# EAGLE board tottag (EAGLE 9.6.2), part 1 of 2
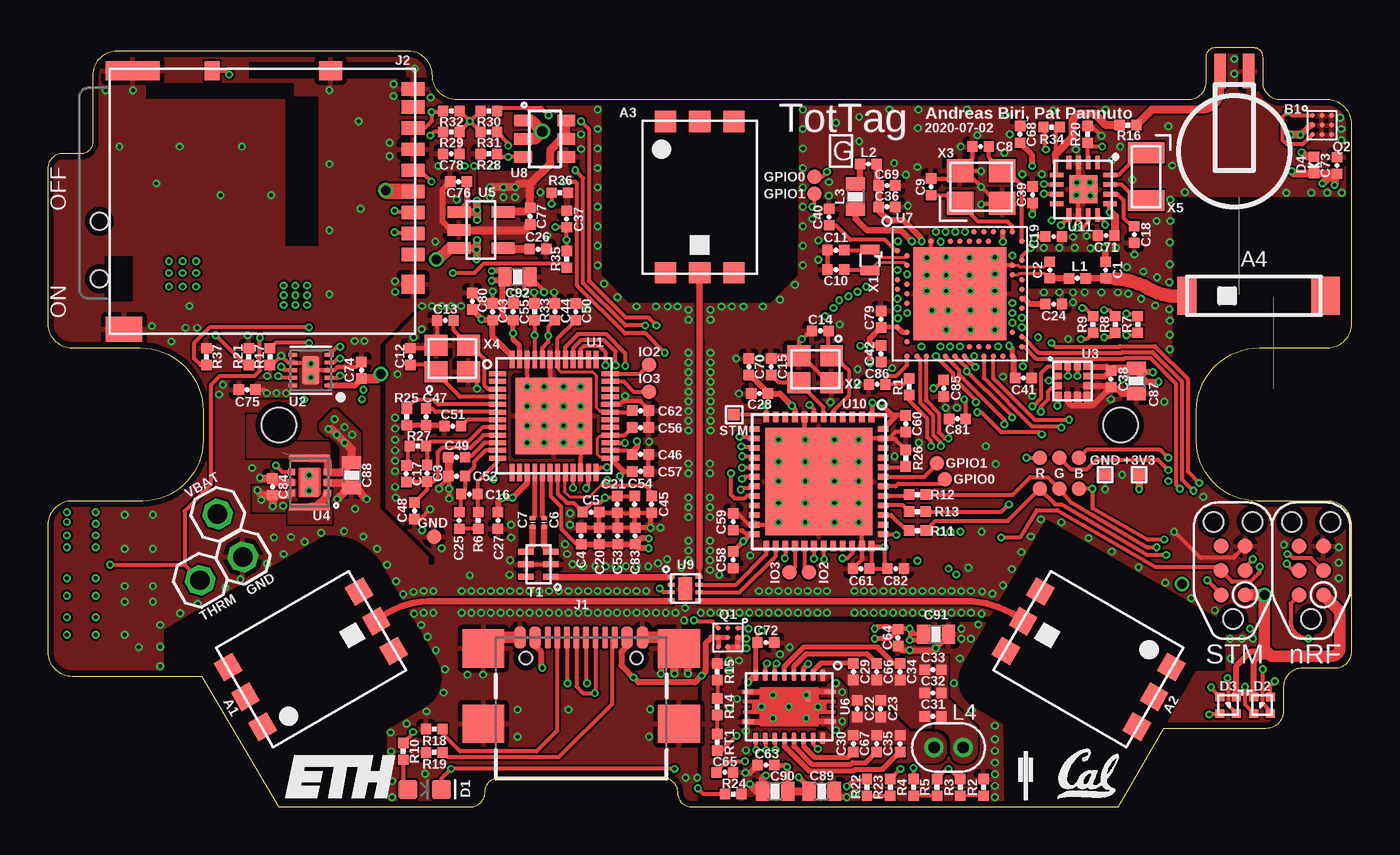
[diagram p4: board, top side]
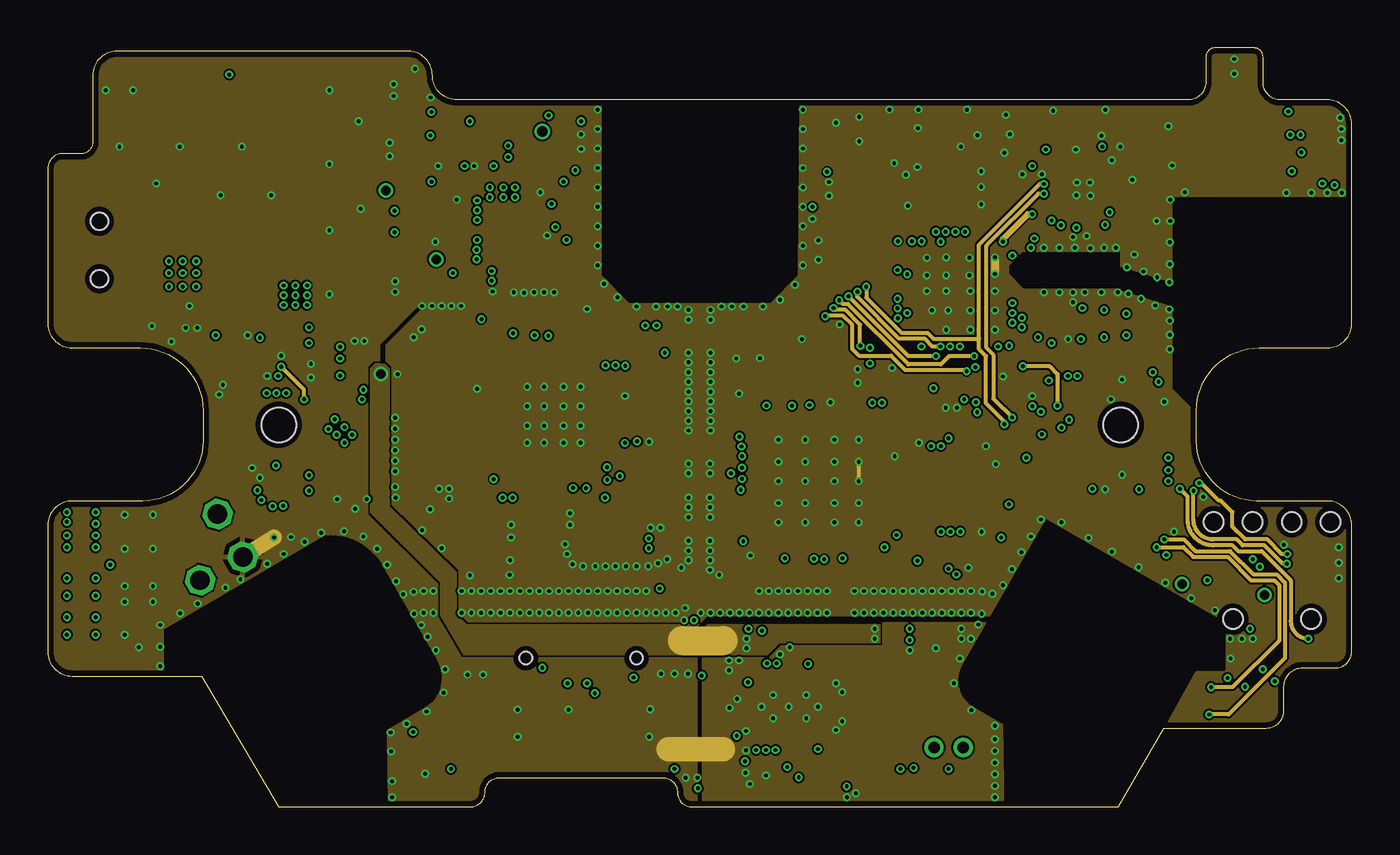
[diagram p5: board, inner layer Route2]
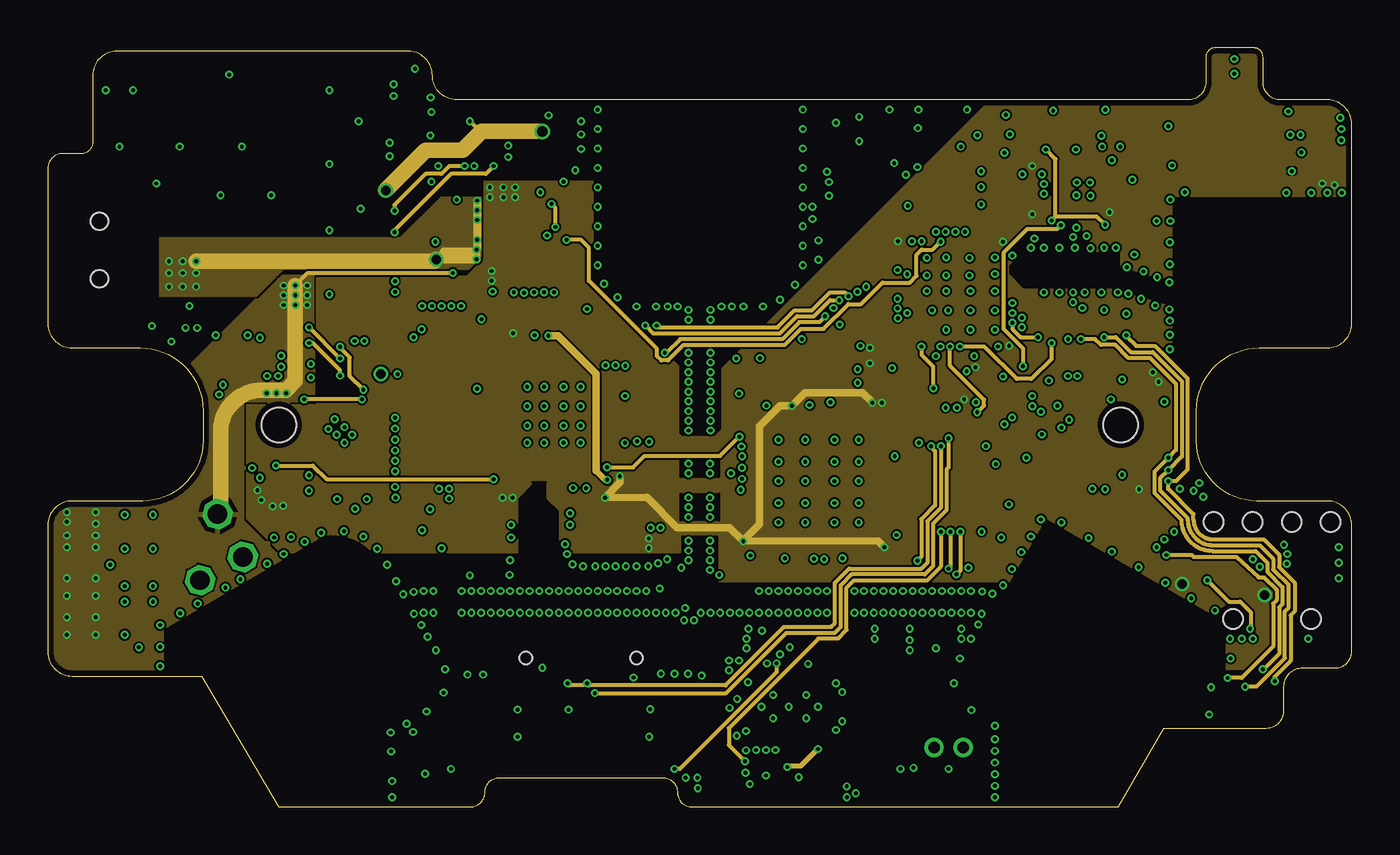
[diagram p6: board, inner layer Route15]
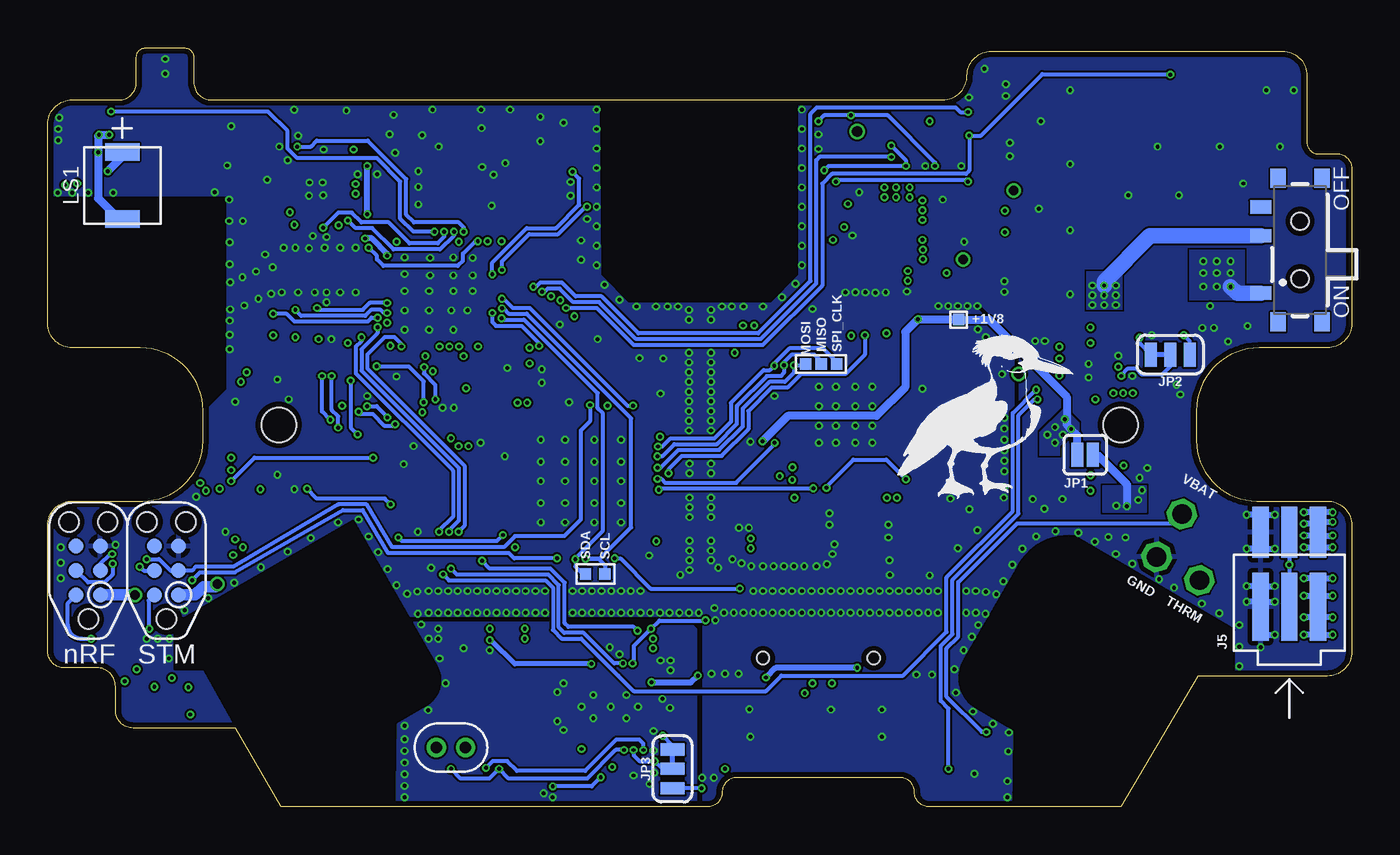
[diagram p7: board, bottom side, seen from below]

Size 68.14 x 39.65 mm. Coordinates in mm from the lower left corner, seen from the top.
Outline: 66.87,36.93 64.42,36.93 arc-90 63.51,37.85 63.51,39.17 arc90 63.02,39.65 60.99,39.65 arc90 60.51,39.17 60.51,37.85 arc-90 59.59,36.93 21.37,36.93 arc-90 20.1,38.2 arc90 18.83,39.47 3.61,39.47 arc90 2.34,38.2 2.34,34.7 arc-90 1.76,34.12 0.76,34.12 arc90 0,33.36 0,25.25 arc90 1.27,23.98 4.83,23.98 arc-90 8.11,20.69 8.11,19.14 arc-90 4.95,15.98 1.27,15.98 arc90 0,14.71 0,8.1 arc90 1.27,6.83 8.03,6.83 12.07,0 22.08,0 arc90 22.84,0.76 arc-90 23.6,1.52 32.14,1.52 arc-90 32.9,0.76 arc90 33.66,0 55.94,0 58.33,4.11 63.68,4.11 arc90 64.6,5.03 64.6,6.3 arc-90 65.56,7.26 67.29,7.26 arc90 68.14,8.11 68.14,14.71 arc90 66.87,15.98 63.18,15.98 arc-90 60.02,19.14 60.02,20.69 arc-90 63.31,23.98 66.87,23.98 arc90 68.14,25.25 68.14,35.66 arc90 66.87,36.93
Copper layers (1+2*15+16): Top 0.0356mm / dielectric 0.18mm / Route2 0.0356mm / dielectric 1.03mm / Route15 0.0356mm / dielectric 0.18mm / Bottom 0.0356mm
Design rules "quickturn_co_kr_1oz_4lyr *": minimum track width 4mil, minimum drill 8mil, track to track 4mil, track to pad 4mil, pad to pad 4mil, via to via 4mil, smd to smd 4mil, copper to edge 12mil, drill to drill 12mil, minimum pad ring 8mil, minimum via ring 4mil, stop-mask expansion 3mil, vias tented up to drill 50mil, thermal gap 10mil
Holes 1.8 mm at 12.07,19.95 56.07,19.95
tKeepout: area 19.3,9.6 to 32.3,11.7; area 34.3,9.6 to 48.8,11.7; area 33.1,12.4 to 35.1,25.7; area 9.7,19.3 to 14.4,20.7; area 53.8,19.3 to 58.3,20.7
tRestrict: area 24.6,13.2 to 26.7,17

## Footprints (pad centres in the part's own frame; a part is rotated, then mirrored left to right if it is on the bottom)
TP06SQ = smd 0.6 x 0.6: TP 0,0
TAIYO-YUDEN-AH086M = smd 1.1 x 1.1: A 0,-3.95; NC0 -1.8,3.95; NC1 0,3.95; NC2 1.8,3.95; NC3 1.8,-3.95; NC4 -1.8,-3.95
AMCA72-2R470G-S1F-T = smd 2 x 1.5: NC 0,3.75 | smd 2 x 1: S1 0,-3.5
MS518SE-FL35E = smd 1.8 x 0.6: + 4.2,0.75; - 4.2,-0.75
0402_CAP = smd 0.536 x 0.546: 1 -0.433,0; 2 0.433,0
0201_CAP = smd 0.3 x 0.21: P$1 0,0.22; P$2 0,-0.22
0603_CAP = smd 0.7 x 1: 1 -0.65,0; 2 0.65,0
LED-0603 = smd 1 x 1: A -0.877,0; C 0.877,0
1MM_SQ_4PAD = smd 0.457 x 0.457: 1 0.432,0.432; 2 0.432,-0.432; 3 -0.432,-0.432; 4 -0.432,0.432
0402_DIODE = smd 0.536 x 0.546: ANODE -0.433,0; CATHODE 0.433,0
PAD.03X.03 = smd 0.762 x 0.762: P$1 0,0
GCT_USB4110-GF-A = smd 0.6 x 1.15: A1/B12 -3.2,1.075; A4/B9 -2.4,1.075; B1/A12 3.2,1.075; B4/A9 2.4,1.075 | smd 0.3 x 1.15: A5 -1.25,1.075; A6 -0.25,1.075; A7 0.25,1.075; A8 1.25,1.075; B5 1.75,1.075; B6 0.75,1.075; B7 -0.75,1.075; B8 -1.75,1.075 | smd 2.18 x 2: S1 -5.11,0.5; S2 5.11,0.5; S3 -5.11,-3.43; S4 5.11,-3.43 | hole 0.65: -2.89,0; 2.89,0
DM3AT-SF-PEJM5 = smd 0.7 x 1.2: 1 3.2,-0.1; 2 2.1,-0.1; 3 1,-0.1; 4 -0.1,-0.1; 5 -1.2,-0.1; 6 -2.3,-0.1; 7 -3.4,-0.1; 8 -4.5,-0.1; B -5.45,-0.1 | smd 1 x 0.8: A -6.4,-10.6 | smd 1 x 1.2: MOUNT0 4.75,-0.1; MOUNT1 -6.4,-4.4 | smd 1 x 2.8: MOUNT2 -6.4,-14.75 | smd 1.3 x 1.9: MOUNT3 7.1,-15.2
TC2030-IDC-NL-2SIDE = smd 0.787 x 0.787: 1 -1.27,-0.635; 2 -1.27,0.635; 3 0,-0.635; 4 0,0.635; 5 1.27,-0.635; 6 1.27,0.635 | smd 0.787 x 0.787 bottom: B1 -1.27,0.635; B2 -1.27,-0.635; B3 0,0.635; B4 0,-0.635; B5 1.27,0.635; B6 1.27,-0.635 | hole 1.016: -2.54,0; 2.54,1.016; 2.54,-1.016
MOLEX-PICO-SPOX-3_SIDE = smd 3.55 x 0.85: 1 -1.725,1.5; 2 -1.725,0; 3 -1.725,-1.5 | smd 2.65 x 0.85: 1SUPP 2.175,1.5; 2SUPP 2.175,0; 3SUPP 2.175,-1.5
1X01 = drill 1.016 octagon: 1 0,0
SMT-JUMPER_2_NO_SILK = smd 0.635 x 1.27: 1 -0.406,0; 2 0.406,0
SMT-JUMPER_3_1-NC_TRACE_SILK = smd 0.635 x 1.27: 1 -1.016,0; 2 0,0; 3 1.016,0
WR222230-26M8-G = drill 0.6: P$1 0,0.762; P$2 0,-0.762
SMT-0440-T-2-R = smd 0.9 x 1.8: + 1.75,0; - -1.75,0
DSBGA = smd 0.25 x 0.25: A1 -0.5,0.5; A2 0,0.5; A3 0.5,0.5; B1 -0.5,0; B2 0,0; B3 0.5,0; C1 -0.5,-0.5; C2 0,-0.5; C3 0.5,-0.5
0402_RES = smd 0.536 x 0.546: 1 -0.433,0; 2 0.433,0
450404015514 = smd 0.7 x 1.1: 1 2.25,-2.05; 2 -0.75,-2.05; 3 -2.25,-2.05 | smd 1 x 0.8: Z1 -3.75,1.15; Z2 3.75,1.15; Z3 3.75,-1.15; Z4 -3.75,-1.15 | hole 0.9: -1.5,0; 1.5,0
EIA-0805 = smd 0.3 x 0.8: 1 -0.65,-0.65; 2 0,-0.65; 3 0.65,-0.65; 4 0.65,0.65; 5 0,0.65; 6 -0.65,0.65
QFN-48-DW1000 = smd 0.9 x 0.26: 1 -2.95,2.2; 2 -2.95,1.8; 3 -2.95,1.4; 4 -2.95,1; 5 -2.95,0.6; 6 -2.95,0.2; 7 -2.95,-0.2; 8 -2.95,-0.6; 9 -2.95,-1; 10 -2.95,-1.4; 11 -2.95,-1.8; 12 -2.95,-2.2; 25 2.95,-2.2; 26 2.95,-1.8; 27 2.95,-1.4; 28 2.95,-1; 29 2.95,-0.6; 30 2.95,-0.2; 31 2.95,0.2; 32 2.95,0.6; 33 2.95,1; 34 2.95,1.4; 35 2.95,1.8; 36 2.95,2.2 | smd 0.26 x 0.9: 13 -2.2,-2.95; 14 -1.8,-2.95; 15 -1.4,-2.95; 16 -1,-2.95; 17 -0.6,-2.95; 18 -0.2,-2.95; 19 0.2,-2.95; 20 0.6,-2.95; 21 1,-2.95; 22 1.4,-2.95; 23 1.8,-2.95; 24 2.2,-2.95; 37 2.2,2.95; 38 1.8,2.95; 39 1.4,2.95; 40 1,2.95; 41 0.6,2.95; 42 0.2,2.95; 43 -0.2,2.95; 44 -0.6,2.95; 45 -1,2.95; 46 -1.4,2.95; 47 -1.8,2.95; 48 -2.2,2.95 | smd 4 x 4: GND 0,0
DSQ0010A = smd 0.5 x 0.2: 1 -0.95,0.8; 2 -0.95,0.4; 3 -0.95,0; 4 -0.95,-0.4; 5 -0.95,-0.8; 6 0.95,-0.8; 7 0.95,-0.4; 8 0.95,0; 9 0.95,0.4; 10 0.95,0.8 | smd 0.9 x 1.5: PAD 0,0
LGA-12 = smd 0.375 x 0.35: 1 -0.75,0.75; 2 -0.75,0.25; 3 -0.75,-0.25; 4 -0.75,-0.75; 7 0.75,-0.75; 8 0.75,-0.25; 9 0.75,0.25; 10 0.75,0.75 | smd 0.35 x 0.375: 5 -0.25,-0.75; 6 0.25,-0.75; 11 0.25,0.75; 12 -0.25,0.75
XCL20X = smd 0.35 x 0.375: 1 -0.55,-0.938; 2 0,-0.938; 3 0.55,-0.938; 4 0.55,0.938; 5 0,0.938; 6 -0.55,0.938 | smd 0.35 x 2.1: 7 -1.275,0; 8 1.275,0 | smd 1.5 x 0.9: PAD 0,0
SOT-23-5 = smd 0.6 x 1.2: 1 -0.95,-1.15; 2 0,-1.15; 3 0.95,-1.15; 4 0.95,1.15; 5 -0.95,1.15
RHL0020A = smd 0.24 x 0.6: 1 -0.775,2.15; 10 -0.775,-2.15; 11 0.775,-2.15; 20 0.775,2.15 | smd 0.6 x 0.24: 2 -1.65,1.75; 3 -1.65,1.25; 4 -1.65,0.75; 5 -1.65,0.25; 6 -1.65,-0.25; 7 -1.65,-0.75; 8 -1.65,-1.25; 9 -1.65,-1.75; 12 1.65,-1.75; 13 1.65,-1.25; 14 1.65,-0.75; 15 1.65,-0.25; 16 1.65,0.25; 17 1.65,0.75; 18 1.65,1.25; 19 1.65,1.75; PAD -0.55,1
AQFN73 = smd 0.3 x 0.3: A8 -1.25,3.25; A10 -0.75,3.25; A12 -0.25,3.25; A14 0.25,3.25; A16 0.75,3.25; A18 1.25,3.25; A20 1.75,3.25; A22 2.25,3.25; A23 2.75,3.25; AA24 3.25,-2.25; AB2 -2.75,-2.5; AC5 -2,-2.75; AC9 -1,-2.75; AC11 -0.5,-2.75; AC13 0,-2.75; AC15 0.5,-2.75; AC17 1,-2.75; AC19 1.5,-2.75; AC21 2,-2.75; AC24 3.25,-2.75; AD2 -2.75,-3.25; AD4 -2.25,-3.25; AD6 -1.75,-3.25; AD8 -1.25,-3.25; AD10 -0.75,-3.25; AD12 -0.25,-3.25; AD14 0.25,-3.25; AD16 0.75,-3.25; AD18 1.25,-3.25; AD20 1.75,-3.25; AD22 2.25,-3.25; AD23 2.75,-3.25; B1 -3.25,2.75; B3 -2.5,2.75; B5 -2,2.75; B7 -1.5,2.75; B9 -1,2.75; B11 -0.5,2.75; B13 0,2.75; B15 0.5,2.75; B17 1,2.75; B19 1.5,2.75; B24 3.25,2.75; C1 -3.25,2.25; D2 -2.75,2; D23 2.75,2; E24 3.25,1.75; F2 -2.75,1.5; F23 2.75,1.5; G1 -3.25,1.25; H2 -2.75,1; H23 2.75,1; J1 -3.25,0.75; J24 3.25,0.75; K2 -2.75,0.5; L1 -3.25,0.25; L24 3.25,0.25; M2 -2.75,0; N1 -3.25,-0.25; N24 3.25,-0.25; P2 -2.75,-0.5; P23 2.75,-0.5; R1 -3.25,-0.75; R24 3.25,-0.75; T2 -2.75,-1; T23 2.75,-1; U1 -3.25,-1.25; U24 3.25,-1.25; V23 2.75,-1.5; W1 -3.25,-1.75; W24 3.25,-1.75; Y2 -2.75,-2; Y23 2.75,-2 | smd 4.85 x 4.85: GND 0,0
TSOT23-6 = smd 0.6 x 0.927: 1 -0.95,-1.126; 2 0,-1.126; 3 0.95,-1.126; 4 0.95,1.126; 5 0,1.126; 6 -0.95,1.126
MLPQ-UT-8 = smd 0.35 x 0.2: 1 -0.725,0.6; 2 -0.725,0.2; 3 -0.725,-0.2; 4 -0.725,-0.6; 5 0.725,-0.6; 6 0.725,-0.2; 7 0.725,0.2; 8 0.725,0.6 | smd 0.7 x 1.2: GND 0,0
UFQFPN-48 = smd 0.55 x 0.3: 1 -3.375,2.75; 2 -3.375,2.25; 3 -3.375,1.75; 4 -3.375,1.25; 5 -3.375,0.75; 6 -3.375,0.25; 7 -3.375,-0.25; 8 -3.375,-0.75; 9 -3.375,-1.25; 10 -3.375,-1.75; 11 -3.375,-2.25; 12 -3.375,-2.75; 25 3.375,-2.75; 26 3.375,-2.25; 27 3.375,-1.75; 28 3.375,-1.25; 29 3.375,-0.75; 30 3.375,-0.25; 31 3.375,0.25; 32 3.375,0.75; 33 3.375,1.25; 34 3.375,1.75; 35 3.375,2.25; 36 3.375,2.75 | smd 0.3 x 0.55: 13 -2.75,-3.375; 14 -2.25,-3.375; 15 -1.75,-3.375; 16 -1.25,-3.375; 17 -0.75,-3.375; 18 -0.25,-3.375; 19 0.25,-3.375; 20 0.75,-3.375; 21 1.25,-3.375; 22 1.75,-3.375; 23 2.25,-3.375; 24 2.75,-3.375; 37 2.75,3.375; 38 2.25,3.375; 39 1.75,3.375; 40 1.25,3.375; 41 0.75,3.375; 42 0.25,3.375; 43 -0.25,3.375; 44 -0.75,3.375; 45 -1.25,3.375; 46 -1.75,3.375; 47 -2.25,3.375; 48 -2.75,3.375 | smd 5.6 x 5.6: GND 0,0
QFN-16-3MM = smd 0.7 x 0.25: 1 -1.4,0.75; 2 -1.4,0.25; 3 -1.4,-0.25; 4 -1.4,-0.75; 9 1.35,-0.75; 10 1.35,-0.25; 11 1.35,0.25; 12 1.35,0.75 | smd 0.25 x 0.7: 5 -0.75,-1.4; 6 -0.25,-1.4; 7 0.25,-1.4; 8 0.75,-1.4; 13 0.75,1.4; 14 0.25,1.4; 15 -0.25,1.4; 16 -0.75,1.4 | smd 1.45 x 1.45: GND 0,0
ABS05 = smd 0.5 x 1: A -0.55,0; B 0.55,0
FA-20H = smd 1.1 x 1.2: 1 -0.7,0.85; 2 -0.7,-0.85; 3 0.7,-0.85; 4 0.7,0.85
TXC-7V = smd 1.4 x 1.2: 1 -1.1,-0.85; 2 1.1,-0.85; 3 1.1,0.85; 4 -1.1,0.85
ABS07 = smd 1.092 x 1.905: 1 -1.245,0; 2 1.245,0

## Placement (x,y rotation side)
+1V8  TPTP06SQ  [TP06SQ]  20.53,25.45 0 bottom
A1  TAIYO-YUDEN-AH086M  [TAIYO-YUDEN-AH086M]  13.75,7.72 120 top
A2  TAIYO-YUDEN-AH086M  [TAIYO-YUDEN-AH086M]  54.39,7.72 240 top
A3  TAIYO-YUDEN-AH086M  [TAIYO-YUDEN-AH086M]  34.07,31.85 0 top
A4  AMCA72-2R47G-S1F-T  [AMCA72-2R470G-S1F-T]  63.02,26.7 270 top
B1  [MS518SE-FL35E]  62.01,34.24 90 top
C1  0.5pF  [0402_CAP]  55.28,28.04 90 top
C2  0.8pF  [0402_CAP]  52.36,28.04 90 top
C3  1.2pF  [0402_CAP]  19.82,17.42 270 top
C4  10pF  [0402_CAP]  27.87,14.15 90 top
C5  10pF  [0402_CAP]  28.38,15.39 0 top
C6  12pF  [0201_CAP]  25.94,14.86 0 top
C7  12pF  [0201_CAP]  25.33,14.86 0 top
C8  12pF  [0402_CAP]  48.75,34.49 0 top
C9  12pF  [0402_CAP]  46.16,32.38 270 top
C10  12pF  [0402_CAP]  41.18,28.07 0 top
C11  12pF  [0402_CAP]  41.18,29.08 0 top
C12  12pF  [0402_CAP]  18.95,23.52 90 top
C13  12pF  [0402_CAP]  20.77,25.41 180 top
C14  12pF  [0402_CAP]  40.37,24.87 180 top
C15  12pF  [0402_CAP]  37.8,22.99 90 top
C16  18pF  [0402_CAP]  22.03,16.33 180 top
C17  27pF  [0402_CAP]  18.73,17.4 270 top
C18  47pF  [0402_CAP]  56.78,29.9 270 top
C19  100pF  [0402_CAP]  52.56,29.79 0 top
C20  330pF  [0402_CAP]  28.81,14.15 90 top
C21  330pF  [0402_CAP]  29.75,15.8 270 top
C22  470pF  [0402_CAP]  42.3,5.13 270 top
C23  470pF  [0402_CAP]  43.52,5.13 270 top
C24  820pF  [0402_CAP]  52.56,26.26 0 top
C25  820pF  [0402_CAP]  21.49,14.96 90 top
C26  10nF  [0402_CAP]  25.61,29.13 0 top
C27  10nF  [0402_CAP]  23.53,14.96 270 top
C28  10nF  [0402_CAP]  37.19,21.59 180 top
C29  10nF  [0402_CAP]  42.09,7.06 270 top
C30  10nF  [0402_CAP]  42.09,3.3 90 top
C31  22nF  [0402_CAP]  46.26,4.72 0 top
C32  22nF  [0402_CAP]  46.26,5.94 0 top
C33  22nF  [0402_CAP]  46.26,7.16 0 top
C34  22nF  [0402_CAP]  44.53,7.06 270 top
C35  22nF  [0402_CAP]  44.53,3.3 90 top
C36  47nF  [0402_CAP]  43.85,31.34 0 top
C37  0.1uF  [0402_CAP]  27.11,30.71 270 top
C38  0.1uF  [0402_CAP]  55.56,22.35 270 top
C39  0.1uF  [0402_CAP]  51.47,31.98 90 top
C40  0.1uF  [0402_CAP]  40.82,30.81 90 top
C41  0.1uF  [0402_CAP]  50.98,22.4 0 top
C42  0.1uF  [0402_CAP]  43.54,23.67 270 top
C43  0.1uF  [0402_CAP]  23.25,25.86 90 top
C44  0.1uF  [0402_CAP]  26.5,25.86 90 top
C45  0.1uF  [0402_CAP]  31.55,15.8 270 top
C46  0.1uF  [0402_CAP]  30.97,18.41 0 top
C47  0.1uF  [0402_CAP]  19.77,20.37 270 top
C48  0.1uF  [0402_CAP]  19.16,15.47 270 top
C49  0.1uF  [0402_CAP]  21.37,18.26 180 top
C50  0.1uF  [0402_CAP]  27.59,25.86 90 top
C51  0.1uF  [0402_CAP]  21.16,19.89 180 top
C52  0.1uF  [0402_CAP]  21.37,17.27 180 top
C53  0.1uF  [0402_CAP]  29.78,14.15 90 top
C54  0.1uF  [0402_CAP]  30.66,15.8 270 top
C55  0.1uF  [0402_CAP]  24.31,25.86 90 top
C56  0.1uF  [0402_CAP]  30.97,19.81 0 top
C57  0.1uF  [0402_CAP]  30.97,17.53 0 top
C58  0.1uF  [0402_CAP]  35.82,12.9 270 top
C59  0.1uF  [0402_CAP]  35.82,14.88 90 top
C60  0.1uF  [0402_CAP]  44.84,20.02 270 top
C61  0.1uF  [0402_CAP]  42.5,12.45 180 top
C62  0.1uF  [0402_CAP]  30.97,20.7 0 top
C63  0.1uF  [0402_CAP]  37.52,2.18 180 top
C64  0.1uF  [0402_CAP]  44.43,8.84 270 top
C65  0.1uF  [0402_CAP]  35.38,1.8 0 top
C66  470nF  [0402_CAP]  43.31,7.06 270 top
C67  470nF  [0402_CAP]  43.31,3.3 90 top
C68  1uF  [0402_CAP]  50.81,35.13 90 top
C69  1uF  [0402_CAP]  43.85,32.46 0 top
C70  1uF  [0402_CAP]  36.63,22.99 90 top
C71  1uF  [0402_CAP]  55.3,29.84 180 top
C72  1uF  [0402_CAP]  37.52,8.59 180 top
C73  1uF  [0402_CAP]  67.37,33.5 90 top
C74  1uF  [0402_CAP]  16.39,22.81 90 top
C75  1uF  [0402_CAP]  10.42,21.79 180 top
C76  4.7uF  [0402_CAP]  21.46,32.66 180 top
C77  4.7uF  [0402_CAP]  25.2,30.86 270 top
C78  4.7uF  [0402_CAP]  21.09,34.11 180 top
C79  4.7uF  [0402_CAP]  43.54,25.48 90 top
C80  4.7uF  [0402_CAP]  22.18,26.42 90 top
C81  4.7uF  [0402_CAP]  47.53,20.27 180 top
C82  4.7uF  [0402_CAP]  44.3,12.45 0 top
C83  4.7uF  [0402_CAP]  30.69,14.15 90 top
C84  4.7uF  [0402_CAP]  11.74,16.71 90 top
C85  4.7uF  [0402_CAP]  46.82,21.87 270 top
C86  4.7uF  [0402_CAP]  43.34,22.07 180 top
C87  10uF  [0603_CAP]  56.88,22.25 270 top
C88  10uF  [0603_CAP]  15.88,17.32 270 top
C89  10uF  [0603_CAP]  40.44,0.81 0 top
C90  10uF  [0603_CAP]  38,0.81 180 top
C91  10uF  [0603_CAP]  46.41,9.02 0 top
C92  47uF  [0603_CAP]  24.54,27.69 0 top
D1  GREEN  [LED-0603]  19.69,0.91 0 top
D2  SML-LX0404SIUPGUSB  [1MM_SQ_4PAD]  63.46,5.31 90 top
D3  SML-LX0404SIUPGUSB  [1MM_SQ_4PAD]  61.68,5.31 0 top
D4  DIODE0402  [0402_DIODE]  66.17,33.53 270 top
GPIO0  TEST-POINT  [PAD.03X.03]  46.87,17.12 0 top
GPIO1  TEST-POINT  [PAD.03X.03]  46.46,17.96 0 top
J1  USB4110-GF-A  [GCT_USB4110-GF-A]  27.87,7.77 0 top
J2  DM3AT-SF-PEJM5  [DM3AT-SF-PEJM5]  19.18,32.05 270 top
J3  TC2030-JLINK-NL-2SIDE  [TC2030-IDC-NL-2SIDE]  66.02,12.34 90 top
J4  TC2030-JLINK-NL-2SIDE  [TC2030-IDC-NL-2SIDE]  61.93,12.34 90 top
J5  MOLEX-PICO-SPOX-3SIDE  [MOLEX-PICO-SPOX-3_SIDE]  3.26,12.17 90 bottom
J6  [1X01]  8.87,15.29 30 top
J7  [1X01]  7.96,11.84 30 top
J8  [1X01]  10.19,13.06 30 top
JP1  JUMPER-SMT_2_NO_SILK  [SMT-JUMPER_2_NO_SILK]  13.93,18.39 180 bottom
JP2  JUMPER-SMT_3_1-NC_TRACE_SILK  [SMT-JUMPER_3_1-NC_TRACE_SILK]  9.48,23.62 180 bottom
JP3  JUMPER-SMT_3_1-NC_TRACE_SILK  [SMT-JUMPER_3_1-NC_TRACE_SILK]  35.49,1.98 90 bottom
L1  4.7nH  [0402_CAP]  53.8,27.61 180 top
L2  15nH  [0402_CAP]  42.88,33.58 180 top
L3  10uH  [0603_CAP]  42.2,31.88 270 top
L4  WR222230-26M8-G  [WR222230-26M8-G]  47.07,3.1 270 top
LS1  PUI_SMT-0440-T-2-R  [SMT-0440-T-2-R]  64.24,32.46 90 bottom
MISO  TPTP06SQ  [TP06SQ]  27.72,23.14 0 bottom
MOSI  TPTP06SQ  [TP06SQ]  28.53,23.14 0 bottom
Q1  CSD75207W15  [DSBGA]  35.54,8.84 270 top
Q2  CSD75207W15  [DSBGA]  66.58,35.61 0 top
R1  4.7  [0402_RES]  45.02,21.95 90 top
R2  97.6  [0402_RES]  48.9,1.02 90 top
R3  97.6  [0402_RES]  47.68,1.02 270 top
R4  162  [0402_RES]  45.24,1.02 270 top
R5  162  [0402_RES]  46.46,1.02 90 top
R6  270  [0402_RES]  22.49,14.96 270 top
R7  1k  [0402_RES]  56.95,25.2 90 top
R8  1k  [0402_RES]  55.78,25.2 90 top
R9  1k  [0402_RES]  54.62,25.2 90 top
R10  1k  [0402_RES]  18.57,2.9 270 top
R11  1k  [0402_RES]  45.45,14.43 180 top
R12  1k  [0402_RES]  45.45,16.31 180 top
R13  1k  [0402_RES]  45.45,15.42 180 top
R14  1k  [0402_RES]  34.98,5.23 270 top
R15  1k  [0402_RES]  34.98,7.06 270 top
R16  1.41k  [0402_RES]  56.45,35.61 0 top
R17  2.2k  [0402_RES]  11.61,23.52 90 top
R18  5.1k  [0402_RES]  20.2,4.06 180 top
R19  5.1k  [0402_RES]  20.2,2.84 180 top
R20  10k  [0402_RES]  54.34,35.13 90 top
R21  10k  [0402_RES]  10.5,23.52 270 top
R22  10k  [0402_RES]  42.81,1.02 270 top
R23  10k  [0402_RES]  44.02,1.02 90 top
R24  10k  [0402_RES]  35.82,0.66 180 top
R25  11k  [0402_RES]  18.75,20.37 90 top
R26  11k  [0402_RES]  44.84,18.21 90 top
R27  16k  [0402_RES]  19.34,18.85 180 top
R28  100k  [0402_RES]  23.04,34.11 180 top
R29  100k  [0402_RES]  21.09,35.26 0 top
R30  100k  [0402_RES]  23.04,36.35 180 top
R31  100k  [0402_RES]  23.04,35.26 180 top
R32  100k  [0402_RES]  21.09,36.35 0 top
R33  100k  [0402_RES]  25.43,25.86 270 top
R34  100k  [0402_RES]  52.46,35.51 180 top
R35  3.3M  [0402_RES]  27.11,28.6 270 top
R36  10M  [0402_RES]  26.75,32.08 180 top
R37  DNP  [0402_RES]  8.29,23.52 270 top
RT1  10k@25C  [0402_RES]  34.98,3.38 270 top
S1  [450404015514]  2.7,29.08 270 bottom
SPI_CLK  TPTP06SQ  [TP06SQ]  26.91,23.14 0 bottom
T1  HHM1595A1  [EIA-0805]  25.64,12.67 90 top
TP1  TPTP06SQ  [TP06SQ]  39.02,12.17 0 bottom
TP2  TPTP06SQ  [TP06SQ]  40.04,12.17 0 bottom
TP3  TPTP06SQ  [TP06SQ]  35.85,20.5 0 top
TP4  TPTP06SQ  [TP06SQ]  55.25,17.35 0 top
TP5  TEST-POINT  [PAD.03X.03]  39.78,12.24 0 top
TP6  TEST-POINT  [PAD.03X.03]  38.77,12.24 0 top
TP7  TEST-POINT  [PAD.03X.03]  52.86,16.61 0 top
TP8  TEST-POINT  [PAD.03X.03]  51.85,16.61 0 top
TP9  TEST-POINT  [PAD.03X.03]  53.88,16.61 0 top
TP10  TEST-POINT  [PAD.03X.03]  20.17,14.1 0 top
TP11  TEST-POINT  [PAD.03X.03]  31.43,23.09 0 top
TP12  TEST-POINT  [PAD.03X.03]  31.43,21.69 0 top
TP13  TEST-POINT  [PAD.03X.03]  40.06,32.92 0 top
TP14  TEST-POINT  [PAD.03X.03]  40.06,32.03 0 top
TP15  TPTP06SQ  [TP06SQ]  57.03,17.35 0 top
TP16  TEST-POINT  [PAD.03X.03]  51.85,18.24 0 top
TP17  TEST-POINT  [PAD.03X.03]  52.86,18.24 0 top
TP18  TEST-POINT  [PAD.03X.03]  53.88,18.24 0 top
U1  DW1000  [QFN-48-DW1000]  26.45,20.42 0 top
U2  BQ24040  [DSQ0010A]  13.75,22.81 180 top
U3  LIS2DW12  [LGA-12]  53.55,22.25 0 top
U4  1.8V  [XCL20X]  13.67,16.94 90 top
U5  MAX8887EZK33+T  [SOT-23-5]  22.63,30.13 270 top
U6  BQ51013B  [RHL0020A]  38.74,5.23 270 top
U7  NRF52840  [AQFN73]  47.66,26.8 0 top
U8  SIP32510  [TSOT23-6]  25.97,34.9 270 top
U9  SKY13317  [MLPQ-UT-8]  33.31,11.4 0 top
U10  STM32F091CC  [UFQFPN-48]  40.29,16.99 270 top
U11  AB1815-T3  [QFN-16-3MM]  54.11,32.26 270 top
U$1  [TOTTERNARY_300MIL]  19.59,16.1 0 bottom
U$2  [UCSD_TRIDENT_SOLID_100MIL]  50.73,0.36 0 top
U$3  [ETH_200MIL]  15.07,0.48 0 top
U$4  [UCB_CAL_100MIL]  52.76,0.46 0 top
X1  32.768kHz  [ABS05]  42.96,28.57 270 top
X2  16MHz  [FA-20H]  40.11,22.86 270 top
X3  32MHz  [TXC-7V]  48.77,32.38 0 top
X4  38.4MHz  [FA-20H]  21.14,23.42 90 top
X5  ABS07-32.768KHZ-7-T  [ABS07]  57.39,32.92 270 top

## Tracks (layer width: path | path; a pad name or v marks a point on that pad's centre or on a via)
!AD_EN  (via drill 0.2)
  Top 0.203: U6.8 37.49,7.41 v37.58,7.49 | v36.61,9.3 36.56,9.34 Q1.A1 | Q1.C1 34.71,9.67 33.9,9.67 33.81,9.75 v33.76,9.75
  Bottom 0.203: v37.58,7.49 37.52,7.55 37.52,8.38 v36.61,9.3 36.18,9.73 33.79,9.73 v33.76,9.75
!CHG  (via drill 0.2)
  Top 0.203: U6.7 37.99,7.4 v38.09,7.49 | D1.C 20.57,1.49 v21.06,1.98 v32.75,1.98 | U2.8 12.38,22.81 v12.2,22.99
  Route2 0.203: v13.39,21.29 13.39,21.79 v12.2,22.99
  Route15 0.203: v38.09,7.49 38.09,7.04 33.03,1.98 v32.75,1.98 | v47.17,14.38 47.17,12.55 v47.07,12.45 | v16.41,21.29 v13.39,21.29
  Bottom 0.203: v38.09,7.49 38.54,7.49 40.14,9.09 41.16,9.09 41.43,9.37 41.43,11.58 41.99,12.14 46.77,12.14 v47.07,12.45 | v21.06,1.98 21.06,5.13 21.47,5.54 21.47,8.41 20.86,9.02 20.86,11.86 17.41,15.32 17.41,20.45 16.57,21.29 v16.41,21.29 | U7.W24 50.91,24.74 51.75,23.9 51.75,22.78 46.67,17.7 46.67,14.95 47.17,14.44 v47.17,14.38
  other vias: 50.91,25.05
!DW_RST  (via drill 0.2)
  Top 0.203: U1.27 v30.15,19.02 v30.15,19.01 | U10.18 36.9,17.26 36.41,17.26 v36.28,17.13
  Bottom 0.203: v30.15,19.01 30.15,18.94 32.17,16.93 35.88,16.93 36.08,17.13 v36.28,17.13
!DW_SPI_CS  (via drill 0.2)
  Top 0.203: U1.24 28.91,17.74 v29.22,17.74 | U10.14 36.59,19.24 36.5,19.33 v36.14,19.33
  Route15 0.203: v29.22,17.74 30.59,17.74 31.19,18.34 35.13,18.34 36.12,19.33 v36.14,19.33
!NRF_CS_IMU  (via drill 0.2)
  Top 0.203: U7.AC11 v47.15,24.05 | U3.2 52.68,22.38 52.53,22.38 52.42,22.27 v52.31,22.27 | v51.95,19.46 51.85,19.56 49.84,19.56 48.79,20.61 v48.56,20.61
  Route15 0.203: v47.15,24.05 47.15,23.05 48.93,21.28 48.93,20.96 48.69,20.73 48.68,20.73 v48.56,20.61
  Bottom 0.203: v52.31,22.27 v52.3,22.26 52.3,19.81 v51.95,19.46
!NRF_CS_RTC  (via drill 0.2)
  Top 0.203: U7.A10 v46.91,30.05 | v52.15,34.34 52.08,34.42 52.08,35.46 R34.2 | U11.12 55.25,30.51 v55.25,30.4
  Route15 0.203: v52.46,30.63 52.66,30.84 | 52.66,30.84 52.66,33.83 v52.15,34.34 | v55.25,30.4 54.82,30.84 52.66,30.84
  Bottom 0.203: v46.91,30.05 46.91,29.84 47.64,29.12 50.08,29.12 51.18,30.23 52.05,30.23 v52.46,30.63
!NRF_CS_SD  (via drill 0.2)
  Top 0.203: v27.57,33.25 27.97,32.84 27.97,27.36 30.18,25.15 v31.22,25.15 | R31.1 24.06,34.67 v24.06,34.54 | J2.2 18.18,29.95 v18.12,30.02
  Route2 0.203: U7.AD16 47.1,23.55 46.67,23.11 44.97,23.11 41.82,26.26 41.56,26.26 v41.36,26.47
  Route15 0.203: v31.22,25.15 31.63,24.74 38.26,24.74 39.15,25.63 40.05,25.63 40.88,26.47 v41.36,26.47 | v23.3,33.48 22.89,33.07 21.06,33.07 18.12,30.12 v18.12,30.02
  Bottom 0.203: v24.06,34.54 23.3,33.78 v23.3,33.48 27.34,33.48 v27.57,33.25
  other vias: 48.41,23.55
!NRF_RST  (via drill 0.2)
  Top 0.203: v64.78,13.21 64.88,13.21 65.09,12.99 66.01,12.99 J3.3 | v52.46,24.23 52.66,24.03 56,24.03 56.04,24.06 57.86,24.06 59.57,22.35 59.57,17.53 v60.18,16.92
  Route2 0.203: v64.78,13.21 64.5,13.21 63.73,13.97 62.57,13.97 61.91,14.64 61.91,15.39 61.3,16 61.19,16 60.28,16.92 v60.18,16.92
  Route15 0.203: U7.AC13 48.93,24.05 50.63,22.35 51.39,22.35 52.46,23.42 v52.46,24.23
  Bottom 0.203: J3.B3 65.39,12.7 64.88,13.21 v64.78,13.21
  other vias: 47.66,24.05
!PG  (via drill 0.2)
  Top 0.203: U2.5 15.12,24.03 v15.27,24.03 | v50.41,25.3 v50.41,25.29
  Route15 0.203: v51.75,24.54 50.83,24.54 50.41,24.96 v50.41,25.29 | v47.68,14.38 47.68,12.34 v47.48,12.14 | v16.49,21.79 15.78,22.5 15.78,23.49 15.27,23.99 v15.27,24.03
  Bottom 0.203: v51.75,24.54 51.75,24.33 52.05,24.03 52.05,22.66 46.97,17.58 46.97,15.15 47.68,14.44 v47.68,14.38 | v47.48,12.14 47.17,11.84 42.13,11.84 41.74,11.45 41.74,9.25 41.28,8.79 40.27,8.79 38.33,6.86 | 38.33,6.86 | 38.33,6.86 37.52,6.05 30.61,6.05 29.8,6.86 23.45,6.86 21.16,9.14 21.16,11.99 17.71,15.44 17.71,20.57 v16.49,21.79
!RTC_IRQ  (via drill 0.2)
  Top 0.203: U11.11 54.36,30.53 54.08,30.25 v53.75,30.25
  Top 0.254: v47.42,30.04 v47.41,30.05 U7.A12
  Bottom 0.203: v47.42,30.04 47.42,29.78 47.77,29.44 49.23,29.44 50.32,30.53 51.75,30.53 52.25,31.04 52.97,31.04 v53.75,30.25
!SD_DETECT  (via drill 0.2)
  Top 0.203: J2.A 9.28,38.45 v9.48,38.25 | R29.1 20.17,35.26 v19.99,35.07
  Route2 0.203: v42.46,24.08 v42.45,24.09 42.45,25.2 41.69,25.96 41.16,25.96 v41.05,26.06
  Bottom 0.203: v9.48,38.25 9.51,38.28 16.17,38.28 19.38,35.07 v19.99,35.07 19.99,34.97 19.98,34.96 19.98,33.24 20.15,33.07 27.16,33.07 27.67,32.56 27.67,27.23 30.77,24.13 37.52,24.13 39.45,26.06 v41.05,26.06 | U7.T2 44.91,25.32 44.71,25.12 43.37,25.12 42.46,24.22 v42.46,24.08
  other vias: 44.91,25.8
!STM_RST  (via drill 0.2)
  Top 0.203: U10.7 40.04,20.76 v39.81,20.99 | J4.3 62.57,12.52 v62.97,12.93
  Bottom 0.203: v39.81,20.99 39.81,20.14 40.29,19.66 40.29,15 41.16,14.14 43.73,14.14 44.3,13.56 50.14,13.56 51.48,15.8 52.97,15.8 58.45,12.55 60.4,12.55 60.6,12.34 J4.B3 61.72,12.34 62.32,12.94 62.82,12.94 62.83,12.93 v62.97,12.93
+1V8  (via drill 0.2)
  Top 0.203: U1.26 29.42,18.6 30.35,18.6 C46.1 30.54,18.53 | U1.48 24.25,23.55
  Top 0.254: v22.66,25.48 22.18,25.96 C80.1
  Top 0.305: 30.54,18.53 30.79,18.79 v30.79,19.09 | 24.25,23.55 23.25,24.55 C43.1 22.74,25.42 C80.1
  Top 0.406: v14.66,19.74 14.83,19.74 15.88,18.68 C88.1 15.4,17.49 U4.3 14.61,18.09 14.48,18.22 U4.8
  Bottom 0.381: 20.56,25.48 +1V8.TP | 14.33,19.41 v14.66,19.74
  Bottom 0.406: 20.56,25.48 v22.66,25.48 23.32,24.81 23.32,21.92 24.82,20.42 29.47,20.42 30.79,19.1 v30.79,19.09 | JP1.2 14.33,19.41 | v14.66,19.74 14.89,19.96 14.89,21.41 18.93,25.45 +1V8.TP
  other vias: 15.91,19.43 14.99,20.24 15.5,19.02 15.09,19.43 15.5,19.84
  pour Top (no thermals): 16.31,19.53 16.31,17.7 15.3,17.7 15.3,18.82 14.76,19.35 14.56,19.35 14.23,19.68 14.23,20.04 14.94,20.75 15.09,20.75
  pour Top (no thermals): 12.63,18.24 12.63,18.03 14.76,18.03 14.76,18.95 14.66,19.05 12.94,19.05 12.83,19.15 12.83,20.47 10.4,20.47 10.4,18.24
  pour Bottom: 15.07,20.78 14.97,20.78 14.26,20.07 14.26,19.66 14.46,19.46 14.66,19.46 15.27,18.85 15.27,18.34 16.29,18.34 16.29,19.56
+3V3  (via drill 0.2, 0.5)
  Top 0.102: U1.28 29.36,19.38 | U1.25 | v36.34,13.88
  Top 0.152: U1.25 29.36,18.26 28.85,18.26 28.72,18.4 28.72,19.25 28.85,19.38 29.36,19.38
  Top 0.203: 44.37,20.45 C60.1 44.12,20.45 | 43.12,20.45 U10.1 43.08,20.41 | U10.36 43.04,12.55 C61.1 C82.1 43.74,12.57 43.74,13.54 v43.73,13.56 | 36.7,14.24 U10.24 36.86,14.29 36.44,14.29 36.28,14.45 C59.1 | U1.19 26.65,16.35 27.12,15.87 27.46,15.87 C5.1 28.42,15.87 28.83,15.87 v29.11,16.15 29.13,16.16 29.68,16.16 C21.1 30.51,16.23 30.59,16.16 C54.1 | C4.1 27.63,13.71 26.84,14.51 26.84,15.66 26.3,16.2 26.3,17.42 U1.18 | 30.09,17.53 C57.1 | C56.1 30.15,19.42 U1.28 | 35.82,13.36 C58.1 | C79.1 43.6,25.05 | v47.89,21.29 47.96,21.21 C81.1 | U7.AD14 48,23.45 48,23.38 48.24,23.14 48.31,23.14 v48.48,22.97 | C70.1 36.71,22.55
  Top 0.254: U10.48 44.37,20.45 | 44.12,20.45 43.59,20.98 v43.59,21.11 | C60.1 43.12,20.45 | 36.7,14.24 v36.34,13.88 35.82,13.36 | U1.25 30.09,17.53 | v29.89,17.28 30.14,17.53 C57.1 | 43.08,20.41 v43.08,21.11 | v38.89,20.96 38.89,20.93 39.03,20.79 U10.9 | U7.Y2 44.66,24.8 U7.W1 43.6,25.05 | U7.AD23 50.41,23.92 v50.23,24.09 | v49.91,29.53 U7.A22 | v44.42,29.55 v44.41,29.55 U7.B1 | v43.73,13.56 43.1,13.56 U10.36 | U1.47 24.64,23.39 24.64,24.1 24.35,24.39 24.31,24.42 v24.31,24.74 C55.1
  Top 0.305: U1.15 25.05,16.91 v24.28,16.15 v23.76,16.15 23.53,15.92 C27.1 | C4.1 C20.1 C53.1 C83.1 | v31.4,13.51 30.89,13.51 C83.1 | C55.1 24,25.42 23.77,25.65 23.77,27.57 C92.1 | v23.2,27.48 23.69,27.48 C92.1 | v23.2,27.99 23.22,28.02 23.56,28.02 C92.1 | U7.AD23 50.45,23.5 50.45,22.5 C41.1 | C39.1 51.47,30.99 v51.44,30.96 | v51.44,33.48 51.42,33.5 51.42,34.09 C68.1 | C79.1 42.96,24.46 v42.96,23.98 | C42.1 43.09,24.11 v42.96,23.98 | v31.4,14.02 31,14.02 C83.1 | U11.13 55.51,31.09 v55.48,31.07 | U3.10 55.34,23 C38.1 55.27,22.5 U3.9 | 36.71,22.55 37.62,21.64 C28.1 38.26,21.59 v38.89,20.96 | v42.96,23.16 v42.96,23.98 | D2.1 63.02,7.57 63.33,7.87 63.94,7.87 | D3.1 62.11,7.37 62.87,8.13 63.68,8.13 | v57.74,22.71 57.07,22.71 C87.1 56.88,22.76 57.44,22.2 v58.05,22.2
  Top 0.381: v57.03,16.59 TP15.TP
  Top 0.406: C71.1 55.76,29.87 55.76,30.84 55.51,31.09 | U8.6 U8.5 26.85,34.9 26.27,34.32 26.27,33.6 25.2,32.54 | C38.1 55.67,22.9 C87.1 | U4.6 12.62,16.28 C84.1 | C84.1 11.21,16.28 v10.95,16.54 | C84.1 v11.74,15.7 | U5.5 25,31.09 C77.1 25.2,32.54 | 25.2,32.54 24.59,32.54 v24.42,32.36 v23.81,32.36 v23.09,32.36 | v65,33.2 65.11,33.09 D4.CATHODE 66.2,33.07 C73.1 | C73.1 67.24,32.94 v67.24,32.49 | C73.1 67.11,33.07 v66.6,32.56
  Top 0.61: J4.1 63.08,11.07 v63.58,11.07 63.58,8.23 63.68,8.13 63.94,7.87 67.09,7.87 arc90 67.52,8.31 67.52,10.21 J3.1
  Route2 0.305: v49.91,29.53 49.91,29.65 51.22,30.96 v51.44,30.96
  Route15 0.203: 43.08,21.13 v43.08,21.11
  Route15 0.381: v36.33,13.89 35.63,14.59 32.88,14.59 31.31,16.17 v29.11,16.15 29.89,16.95 v29.89,17.28 | v43.73,13.56 43.4,13.88 v36.33,13.89 | v36.33,13.89 v36.34,13.88 | v36.33,13.89 37.19,14.77 37.19,19.89 38.26,20.96 v38.89,20.96 v38.9,20.96 39.58,21.64 42.57,21.64 43.08,21.13 | v36.33,13.89
  Bottom 0.203: v48.48,22.97 48.48,22.64 47.89,22.05 v47.89,21.29
  Bottom 0.305: v51.44,30.96 v51.44,33.48
  Bottom 0.406: v11.74,15.7 11.74,16.84 13.29,18.39 JP1.1 | v65,33.2 64.24,33.96 LS1.+
  Bottom 0.61: J3.B1 v63.58,11.07 | J4.B1 60.43,11.07 60,11.51 59.39,11.51 v59.27,11.63
  other vias: 11.16,16.03 12.3,15.72 23.1,31.85 23.81,31.85 24.42,31.85
  pour Route15 (rank 2): 14.05,27.69 14.05,20.98 10.4,20.98 10.4,15.09 12.17,13.31 33.05,13.31 33.05,14.25 35.08,14.25 35.08,11.79 55.5,11.79 60,7.21 67.98,7.21 67.98,15.33 67.3,15.98 59.91,15.98 59.9,15.98 59.95,20.55 arc-90 63.43,24.03 67.09,24.03 arc90 68.1,25.04 68.1,32.66 68.05,32.66 68.05,36.53 64.27,40.31 60.86,40.31 57.49,36.93 49.28,36.93 35.24,22.89 35.24,19.71 34.84,19.3 33.15,19.3 32.95,19.5 32.95,23.01 28.48,27.48 28.48,32.66 22.79,32.66 22.79,28.6 21.88,27.69
  pour Top (rank 2, no thermals): 13.01,16.74 13.01,15.42 10.73,15.42 10.73,16.74
  pour Bottom (rank 2, no thermals): 13.01,16.74 13.01,15.42 10.73,15.42 10.73,16.74
  pour Top (no thermals): 22.49,32.87 22.49,31.85 22.79,31.55 22.89,31.55 24.62,31.55 24.92,31.85 25.53,31.85 25.53,33.17 22.49,33.17
  cutout Top: 68.61,20.27 60.38,20.27 58.81,21.84 58.81,31.85 68.61,31.85
  cutout Bottom: 69.22,20.27 60.38,20.27 58.81,21.84 58.81,31.85 69.22,31.85
  cutout Route15: 69.02,20.27 60.38,20.27 58.81,21.84 58.81,31.85 69.02,31.85
  cutout Route2: 68.82,20.27 60.38,20.27 58.81,21.84 58.81,31.85 68.82,31.85
  cutout Route15: 64.75,33.17 64.75,33.27 64.75,33.38 64.85,33.48 65.16,33.48 65.26,33.38 65.26,33.07 65.16,32.97 64.85,32.97 64.75,33.07
ANT_SEL1  (via drill 0.2)
  Top 0.152: U9.3 32.66,11.2
  Top 0.203: U10.27 38.54,13.01 v38.51,12.98 | v31.97,11.4 32.18,11.2 32.66,11.2
  Bottom 0.203: v38.51,12.98 38.21,12.98 36.63,11.4 v31.97,11.4
ANT_SEL2
  Top 0.203: U9.6 36.15,11.2 38.04,13.09 U10.26
ANT_SEL3
  Top 0.203: U10.25 37.54,13.19 35.97,11.61 33.95,11.61 U9.7
BATIN  (via drill 0.2)
  Top 0.203: U7.B9 v46.66,29.53 | v26.52,30.29 26.54,30.28 C37.2 v27.11,29.62 R35.1 | R36.2 v26.32,31.5
  Route15 0.203: v46.66,29.53 46.24,29.11 45.66,29.11 45.4,28.84 45.4,27.74 45.04,27.38 43.62,27.38 42.5,26.26 41.83,26.26 40.54,24.97 39.35,24.97 38.51,24.13 33.23,24.13 32.42,23.32 32.06,23.32 31.83,23.55 31.83,23.93 28.28,27.48 28.28,29.21 27.87,29.62 v27.11,29.62 | v26.52,30.29 26.52,31.29 v26.32,31.5
BATT_THERM  (via drill 0.2)
  Top 0.203: v11.08,24.51 11.08,22.78 10.79,22.5 8.99,22.5 8.52,22.02 8.52,16.83 7.14,15.45 7.14,12.65 | 7.14,12.65 J7.1 | v3.26,12.65 7.14,12.65
  Bottom 0.203: J5.2SUPP v3.26,12.65 J5.2 | JP2.3 11.08,24.21 v11.08,24.51
BATT_TS  (via drill 0.2)
  Top 0.203: U2.9 12.13,22.41 v12.04,22.5
  Bottom 0.203: v12.04,22.5 12.04,22.56 11.68,22.91 11.28,22.91 10.98,22.61 9.89,22.61 9.48,23.01 JP2.2
BLE_ANT
  Top 0.33: L1.1 C1.1
  Top 0.61: C1.1 55.81,27.58
  Top 0.711: 55.81,27.58 arc-28 57.54,27.08 arc39 A4.S1
BQ_AC1
  pour Top (rank 2, no thermals): 46.16,7.87 46.16,4.11 45.14,4.11 44.02,5.23 41.48,5.23 41.48,6.53 40.27,6.53 40.27,7.87
BQ_AC2
  pour Top (rank 2, no thermals): 40.27,2.29 40.27,3.96 41.48,3.96 41.48,5.03 43.92,5.03 45.04,3.91 46.26,3.91 arc-90 46.97,3.2 46.97,2.9 arc-90 46.26,2.29
BQ_BOOT1
  Top 0.254: U6.3 39.99,7.09 40.42,7.52 42.07,7.52 C29.1
BQ_BOOT2
  Top 0.254: U6.17 39.49,3.16 40.06,2.59 41.82,2.59 C30.1
BQ_CLAMP1
  Top 0.254: U6.5 38.99,7.34 39.66,8 42.81,8 C66.1
BQ_CLAMP2
  Top 0.254: U6.16 38.99,3.16 39.91,2.24 41.97,2.24 42.05,2.31 42.76,2.31 C67.1
BQ_COMM1
  Top 0.254: U6.6 38.49,7.34 39.51,8.36 43.31,8.36 44.18,7.49 C34.1
BQ_COMM2
  Top 0.254: C35.1 43.62,1.96 42.2,1.96 42.12,1.88 39.77,1.88 38.49,3.15 U6.15
BQ_FOD  (via drill 0.2)
  Top 0.152: R3.1 47.6,1.45 v47.07,1.98
  Top 0.203: U6.14 37.99,3.01 v38.03,2.97 | v44.56,1.98 R23.2 | R5.2 46.99,1.98 v47.07,1.98
  Bottom 0.203: v38.03,2.97 38.46,2.97 39.96,1.47 44.05,1.47 v44.56,1.98 45.07,1.47 46.56,1.47 v47.07,1.98
BQ_ILM  (via drill 0.2)
  Top 0.203: U6.12 36.99,2.99 v37.01,2.97 | v45.24,2.03 R4.1
  Bottom 0.203: v37.01,2.97 37.01,3.3 37.22,3.51 38.44,3.51 40.06,1.88 43.62,1.88 44.13,2.39 44.89,2.39 v45.24,2.03
BQ_RECT  (via drill 0.2)
  Top 0.203: v41.75,1.07 42.05,1.37 42.73,1.37 R22.1 | U6.18 39.99,3.27 v40.24,3.02
  Top 0.254: C63.1 38.54,2.18 v38.64,2.08 38.66,2.07 C90.1 | C89.1 39.79,0.99 v39.24,1.54
  Top 0.406: C90.1 C89.1
  Route15 0.254: v38.64,2.08 38.68,2.13 39.34,2.13 v40.24,3.02
  Bottom 0.203: v39.24,1.54 39.72,1.07 v41.75,1.07
BUZZER_GATE  (via drill 0.2)
  Top 0.203: U7.A14 v47.93,30.05 | Q2.A1 65.04,36.11 v64.83,36.32 64.52,36.02 64.52,34.85 64.77,34.6 65.57,34.6 Q2.C1
  Bottom 0.203: v47.93,30.05 49.03,30.05 49.71,30.73 49.71,32.66 50.93,33.88 55.1,33.88 55.61,34.39 55.61,35.31 56.62,36.32 v64.83,36.32
COIL_AC1
  pour Top (no thermals): 46.36,7.87 46.36,4.11 arc-90 47.17,3.3 47.17,2.9 arc90 47.78,2.29 47.89,2.29 arc90 48.6,3 48.6,4.11 47.07,5.64 47.07,7.87
D+  (via drill 0.2)
  Top 0.203: U7.AD6 45.88,23.52 45.88,21.26 46.56,20.57 46.56,19.56 46.87,19.25 v47.07,19.25 | J1.B6 28.62,5.98 v28.58,5.94 27.97,5.94 27.62,6.3 J1.A6
  Route15 0.203: v28.58,5.94 35.44,5.94 38.59,9.09 41.13,9.09 41.43,9.4 41.43,11.57 42,12.14 45.83,12.14 46.26,12.57 46.26,14.78 46.97,15.49 46.97,17.63 47.07,17.73 v47.07,19.25
D-  (via drill 0.2)
  Top 0.203: U7.AD4 45.57,23.38 45.57,21.13 46.26,20.45 46.26,19.43 46.67,19.03 v46.67,18.85 | J1.B7 27.12,6.49 v27.16,6.45 | J1.A7 28.12,6.51 v28.17,6.45
  Route15 0.203: v27.16,6.45 27.26,6.35 28.28,6.35 | 28.28,6.35 35.41,6.35 38.46,9.4 40.93,9.4 41.13,9.6 41.13,11.7 41.88,12.45 45.65,12.45 45.95,12.75 45.95,14.91 46.67,15.62 v46.67,18.85 | v28.17,6.45 28.28,6.35
DW_IRQ  (via drill 0.2)
  Top 0.203: U1.45 25.45,24.44 25.44,24.44 v25.44,24.64 25.44,25.41 R33.2 | U10.20 36.54,16.24 36.41,16.1 35.9,16.1 35.69,16.31 v35.69,17.42
  Bottom 0.203: v25.44,24.64 25.44,23.62 26.46,22.61 28.78,22.61 29.5,21.89 30.31,21.89 31.53,20.68 31.53,19.74 32.92,18.34 34.98,18.34 35.69,17.63 v35.69,17.42
DW_SPI_CLK  (via drill 0.2)
  Top 0.203: U1.41 27.05,24.03 27.7,24.69 29.18,24.69 30.17,23.7 v30.17,23.04 | v36.25,18.83 36.35,18.83 36.39,18.79 36.86,18.79 U10.15
  Bottom 0.203: v36.25,18.83 36.02,18.83 35.59,19.25 33.3,19.25 32.44,20.12 32.44,21.1 30.73,22.81 30.4,22.81 v30.17,23.04 30.17,23.16 29.39,23.95 27.64,23.95 26.9,23.21 SPI_CLK.TP
DW_SPI_MISO  (via drill 0.2)
  Top 0.203: U1.40 27.46,23.39 27.46,23.98 27.87,24.38 29.06,24.38 29.67,23.77 v29.67,23.06 | v36.28,18.32 36.31,18.29 36.86,18.29 U10.16
  Bottom 0.203: v36.28,18.32 36.02,18.32 35.39,18.95 33.18,18.95 32.14,19.99 32.14,20.95 32.12,20.95 30.56,22.5 29.83,22.5 29.67,22.67 v29.67,23.06 29.67,23.21 29.24,23.64 28.09,23.64 27.72,23.27 MISO.TP
DW_SPI_MOSI  (via drill 0.2)
  Top 0.203: U1.39 27.86,23.39 27.86,23.93 28.01,24.08 28.81,24.08 29.14,23.75 v29.14,23.06 | v36.28,17.71 v36.28,17.72 36.89,17.72 U10.17
  Bottom 0.203: MOSI.TP 28.61,23.06 v29.14,23.06 29.14,22.68 29.62,22.2 30.43,22.2 31.83,20.8 31.83,19.86 33.05,18.64 35.19,18.64 36.12,17.71 v36.28,17.71
DW_WAKEUP  (via drill 0.2)
  Top 0.203: 28.24,17.46 28.24,16.75 v28.13,16.65 | U10.19 36.71,16.74 36.64,16.67 36.31,16.67 v36.21,16.56 | U1.23 28.24,17.46 | 28.24,17.46
  Bottom 0.203: v28.13,16.65 28.16,16.62 36.27,16.62 v36.21,16.56 | v36.21,16.56
EXT_I2C_SCL  (via drill 0.2)
  Top 0.203: U10.30 v40.04,12.95 | v44.41,26.04 v44.41,26.05
  Bottom 0.203: v44.41,26.04 44.33,26.04 44.05,25.76 43.12,25.76 37.65,20.29 37.65,14.6 39.3,12.95 v40.04,12.95 39.35,12.95 39.02,12.62 TP1.TP
EXT_I2C_SDA  (via drill 0.2)
  Top 0.203: U10.31 40.54,12.96 v40.57,12.93 | U7.U1 v44.42,25.53
  Bottom 0.203: v44.42,25.53 44.34,25.45 43.25,25.45 39.4,21.61 39.4,20.83 39.13,20.56 39.13,14.44 40.57,13 v40.57,12.93 40.57,12.55 40.19,12.17 TP2.TP
GND  (via drill 0.2)
  Top 0.102: 47.4,27.43 47.4,27.05 U7.GND 45.93,28.52 v45.93,28.68
  Top 0.152: U1.GND 25.3,21.56 | U1.GND v27.85,19.02 | U1.GND v27.84,19.02 | U7.F23 50.69,28.3 50.77,28.22 52.1,28.22 C2.2
  Top 0.203: 43.92,19.21 43.7,19.21 U10.47 42.67,19.24 | 43.92,19.21 44.29,19.58 C60.2 | R26.2 44.27,19.21 43.92,19.21 | 40.55,16.74 42.54,14.74 U10.35 42.54,12.92 C61.2 | 40.55,16.74 40.35,16.93 | 40.55,16.74 38.55,14.74 U10.23 36.65,14.74 36.07,15.32 C59.2 | U10.8 39.54,17.74 | U10.8 39.57,20.4 U10.8 | 42.67,19.24 40.35,16.93 | U1.43 26.25,20.62 | 26.25,20.62 U1.GND | U1.46 25.05,21.82 25.3,21.56 26.25,20.62 | v27.85,19.02 U1.22 | T1.5 T1.2 | C53.2 C83.2 30.69,15.34 | C53.2 C20.2 | C20.2 C4.2 C20.2 | C20.2 C5.2 | C5.2 | C53.2 29.77,15.34 | 29.77,15.34 C21.2 28.84,15.37 C5.2 | 30.69,15.34 C54.2 C45.2 | 29.77,15.34 30.69,15.34 | C57.2 C46.2 | C56.2 C62.2 | 31.31,20.7 C62.2 | U1.32 29.88,21.02 30.04,21.18 30.96,21.18 31.4,20.73 C62.2 | C5.2 | X2.2 39.26,24.3 v39.4,24.43 39.83,24.87 C14.2 | X2.4 40.8,22.16 39.71,23.24 39.73,23.24 39.42,23.56 X2.2 | U10.8 39.54,17.74 | 39.54,17.74 U10.GND | C5.2 | C20.2 C5.2 | C5.2 28.91,15.49 C5.2 | C20.2 C5.2 | C20.2 C5.2 | C5.2 | 39.54,17.74 U10.GND | U10.8 39.54,17.74 | C20.2 C5.2 | C20.2 C5.2 | C5.2 | 40.35,16.93 U10.GND | 40.35,16.93 | C53.2 C20.2 | U10.8 39.54,17.74 | 39.54,17.74 U10.GND | 42.67,19.24 40.35,16.93 | U7.F23 48.7,28.3 48.55,28.45 47.66,27.56 47.66,27.18 | 47.66,27.18 U7.GND | U7.B7 46.16,28.68 47.4,27.43 47.66,27.18 | C11.1 C10.1 | C13.2 20.34,24.17 X4.4 20.12,23.95 C12.2 | v19.97,15.54 19.46,15.04 C48.2 | C80.2 22.74,26.29 C43.2 v23.25,26.92 | v25.41,26.87 25.43,26.85 R33.1 | v26.45,26.87 26.45,26.34 C44.2 | C50.2 27.89,26.29 v28.17,26.01 | v22.43,21.84 22.43,22.27 X4.2 | C8.1 48.32,33.88 X3.4 | C9.1 47.26,32.82 X3.4 | v48.77,31.47 49.81,31.47 X3.2 49.62,31.53 v48.77,32.38 47.92,33.23 X3.4 | v20.96,16.1 v20.96,16.61 20.96,17.25 C52.2 20.93,17.17 20.45,16.69 v20.45,16.61
  Top 0.203: U11.10 53.86,31.85 v53.75,31.95 | v13.75,22.43 14.13,22.81 U2.3 14.97,22.81 15.14,22.99 16.13,22.99 C74.2 | v13.75,23.14 13.68,23.21 U2.7 12.56,23.21 v12.2,23.57 11.71,23.09 R17.1 | U6.PAD 39.69,5.78 v39.63,5.84 | R20.2 54.54,35.56 v55.05,35.05 | X2.2 37.94,23.56 C15.2 | v48.77,33.2 47.71,33.2 X3.4 | v24.35,26.87 24.35,26.33 C55.2 | v24.89,26.86 24.89,27.38 C92.2 25.93,26.95 v25.93,26.89 | J4.5 61.96,13 60.23,13 v58.86,14.38
  Top 0.254: C51.2 20.68,19.94 C47.2 R25.1 | C83.2 v31.5,14.58 31.5,15.31 C45.2 | U11.3 53.86,32.69 v53.78,32.61 53.78,32.59 U11.GND | C91.2 47.06,8.93 v46.41,8.28
  Top 0.305: U6.10 37.74,6.01 v37.9,5.84 | U6.11 37.74,4.46 v37.9,4.62 | U6.20 39.8,4.46 v39.63,4.62 | C90.2 37.06,0.81 | v36.46,1.78 36.68,1.78 C63.2 | v41.75,0.51 41.4,0.51 C89.2 | U6.1 39.97,6.01 U6.PAD | U3.5 53.3,21.15 53.47,20.98 53.98,20.98 | 53.98,20.98 54.49,20.98 | U3.6 53.8,21.16 53.98,20.98 | U3.7 54.3,21.17 54.49,20.98 | J1.S2 32.04,7.33 v32.04,6.96 | 54.49,20.98 54.62,20.98 C38.2 | C38.2 55.79,21.92 56.11,21.59 56.87,21.59 C87.2 | U3.8 55.47,22 C38.2 | U5.2 21.05,30.13 20.63,30.56 20.63,32.26 C76.2 | C64.2 44.66,8.18 v45.04,8.18 46.31,8.18 v46.41,8.28
  Top 0.33: C1.2 55.28,29.06 55.2,29.13 v55.2,29.21
  Top 0.406: 37.06,0.81 v36.68,1.19 | U4.5 11.95,16.94 C84.2 11.13,17.15 v11.08,17.2 | C49.2 C52.2 | U4.2 15.61,16.94 C88.2 | C88.2 16.07,16.67 v16.67,16.08 | C88.2 15.71,16.67 v15.12,16.08 | U5.2 24.91,30.13 C77.2 | v32.75,6.96 32.75,8.04 J1.S2 33.46,7.79 v33.46,6.96 | v37.52,1.64 37.35,1.47 C90.2
  Top 0.61: J1.B1/A12 32.41,8.85 J1.S2 | J1.A1/B12 23.33,8.85 J1.S1
  Route2 0.203: v42.37,18.03 v42.37,17.02
  Route2 0.406: v49.49,28.7 v49.49,27.84
  Route2 0.813: J8.1 v11.82,14.07
  Route2 1.27: 32.44,3 35.29,3
  Bottom 0.305: J5.1 4.76,8.99 v4.02,8.99 | 4.76,10.72 v4.02,10.72 | 4.76,11.53 v4.02,11.53 | J5.1 4.76,11.53 | 4.76,11.53 v5.49,11.53 | J5.1 4.76,10.72 | 4.76,10.72 v5.49,10.72 | 4.76,13.49 v4.02,13.49 | 4.76,15.27 v4.02,15.27 | 4.76,15.27 J5.1SUPP 4.76,13.49 | 4.76,15.27 v5.49,15.27 | 4.76,13.49 v5.49,13.49
  other vias: 19.11,11.23 20.15,11.28 21.62,11.28 22.13,11.28 22.64,11.28 23.15,11.28 23.65,11.28 24.16,11.28 24.67,11.28 25.18,11.28 25.69,11.28 26.19,11.28 26.7,11.28 27.21,11.28 27.72,11.28 28.23,11.28 28.73,11.28 29.24,11.28 29.75,11.28 30.26,11.28 30.77,11.28 31.27,11.28 32.37,12.93 31.88,12.73 33.1,12.5 33.48,12.88 33.48,13.39 33.48,13.89 33.48,15.14 33.48,15.65 33.48,16.15 33.48,17.42 33.48,17.93 33.48,19.66 34.63,19.66 34.6,17.42 33.48,22.2 33.48,22.71 33.48,23.22 33.48,23.72 34.63,23.72 34.63,23.22 34.63,22.71 34.63,22.2 34.63,21.69 34.63,21.18 34.6,16.15 34.6,15.65 34.6,15.14 34.6,13.89 34.6,13.39 34.6,12.88 34.6,12.37 35.08,12.12 37.67,11.28 38.18,11.28 38.69,11.28 39.2,11.28 39.71,11.28 40.21,11.28 40.72,11.28 42.15,11.28 43.67,11.28 44.18,11.28 44.69,11.28 45.19,11.28 45.7,11.28 46.21,11.28 46.72,11.28 47.23,11.28 47.73,11.28 48.24,11.28 27.84,21.95 25.94,21.95 25.05,21.95 25.05,20.93 25.94,20.93 26.96,21.95 27.84,20.93 26.96,20.93 27.84,19.91 26.96,19.02 25.94,19.02 25.05,19.02 25.05,19.91 25.94,19.91 26.96,19.91 38.18,19.18 39.58,19.18 41.1,19.18 42.37,19.18 41.1,18.03 38.18,18.03 41.1,17.02 39.58,17.02 39.58,15.88 39.58,14.86 38.18,14.86 41.1,14.86 42.37,14.86 42.37,15.88 41.1,15.88 38.18,15.88 36.13,21.59 18.57,11.1 19.13,10.08 20.15,10.13 21.62,10.13 22.13,10.13 22.64,10.13 23.15,10.13 23.65,10.13 24.16,10.13 24.67,10.13 25.18,10.13 25.69,10.13 26.19,10.13 26.7,10.13 27.21,10.13 27.72,10.13 28.23,10.13 28.73,10.13 29.24,10.13 29.75,10.13 30.26,10.13 30.77,10.13 31.27,10.13 31.78,10.13 32.29,10.13 32.8,10.13 33.31,10.39 34.12,10.13 34.63,10.13 35.13,10.13 35.64,10.13 36.15,10.13 36.66,10.13 37.17,10.13 37.67,10.13 38.18,10.13 38.69,10.13 39.2,10.13 39.71,10.13 40.21,10.13 40.72,10.13 43.67,10.13 44.18,10.13 44.69,10.13 45.19,10.13 45.7,10.13 46.21,10.13 46.72,10.13 47.23,10.13 47.73,10.13 48.24,10.13 19.56,14.45 18.27,22.61 27.13,13.21 45.52,19.02 39.58,18.03 38.18,17.02 18.19,11.79 19.51,9.5 19.84,8.89 48.62,9.53 48.24,8.79 49.36,11.13 50.37,12.42 49.92,11.58 33.48,25.45 32.9,26.14 32.39,26.14 34.63,25.45 35.21,26.14 35.74,26.14 48.83,11.25 48.8,10.08 18.14,27.46 19.11,24.54 18.14,19.76 21.93,6.91 42.15,10.13 45.93,26.95 47.05,25.93 48.22,25.93 49.49,25.93 45.93,27.76 46.95,28.7 46.95,27.76 49.49,26.95 48.22,26.95 14.28,14.33 16.49,14.12 15.48,14.4 53.58,26.37 52.86,26.87 52.05,26.87 45.45,33.43 41.38,25.2 35.97,23.42 40.9,21.13 36.71,13.13 20.07,26.16 18.14,26.9 20.58,26.16 53.32,24.43 49.54,17.91 49.03,18.85 48.11,12.5 49.92,22.48 48.8,14.38 51.37,14.12 51.9,15.01 39.05,27.28 42.4,36.04 45.47,35.46 58.63,24.66 44.25,18.31 50.88,13.31 20.28,8.18 20.76,7.19 20.68,5.97 19.79,4.98 33.26,9.75 17.74,12.65 17.2,13.49 31.43,3.66 47.35,6.45 47.66,7.75 56.14,17.35 20.4,33.48 20.58,13.51 27.03,13.72 24.54,3.66 48.27,5.05 27.41,12.67 27.97,12.57 28.61,12.57 29.14,12.57 29.67,12.57 30.21,12.57 30.77,12.57 31.38,12.57 24.14,12.12 22.05,12.09 24.16,12.88 24.21,14.73 24.21,14.07 18.14,20.32 19.54,24.94 55.25,16.59 53.58,26.87 55.05,26.87 52.05,29.21 52.86,29.21 53.68,29.21 56.39,28.19 57.87,26.19 54.49,29.18 49.99,34.16 55.81,29.21 47.71,34.49 41.18,35.74 54.46,32.61 54.49,31.93 43.97,36.42 53.73,34.34 52.53,36.37 48.04,36.42 45.5,36.42 58.63,29.49 58.55,35.56 55.26,36.42 56.04,34.49 54.18,26.87 58.6,27.41 58.6,25.98 13.42,13.84 12.33,13.21 11.46,12.7 10.06,11.89 9.28,11.46 7.83,10.62 6.92,10.11 5.87,9.5 5.87,7.34 5.87,8.36 20.25,29.51 21.37,31.72 25.74,32.11 26.09,29.84 36.35,26.14 37.37,26.14 31.78,26.14 30.77,26.14 29.78,26.62 29.06,27.33 28.73,36.42 28.73,35.41 28.73,34.39 28.73,33.38 28.73,32.36 28.73,31.34 28.73,30.33 28.73,29.31 28.73,28.3 62.01,39.07 67.47,13.56 61.78,8.79 52.97,14.86 54.39,14.05 55.61,13.34 57,12.52 58.4,11.71 61.8,7.75 60.99,10.26 59.75,10.9 46.95,24.92 48.22,24.92 49.49,24.92 58.76,33.5 59.42,32.11 58.63,28.35 57.97,27.66 51.95,33.05 38.26,26.49 44.23,33.63 22.28,33.48 39.45,36.42 39.45,35.41 39.45,34.39 39.45,33.38 39.45,32.36 39.45,31.34 39.45,30.33 39.45,29.31 39.45,28.3 44.84,33.02 44.94,31.39 46.95,26.95 46.21,25.93 34.6,17.93 33.48,21.69 33.48,21.18 33.48,20.68 33.48,20.17 34.63,20.68 34.63,20.17 33.48,25.96 34.63,25.96 40.27,28.57 40.27,29.59 40.82,31.93 42.4,34.77 48.16,27.76 48.16,28.68 18.07,37.74 19.18,38.56 17.86,34.7 17.86,33.99 30.16,21.46 4.45,37.44 3.03,37.44 4.76,8.33 6.46,24.31 31.48,5.11 27.87,34.37 27.87,35.13 20,37.06 18.07,37.13 31.43,19.08 27.29,14.73 27.29,15.34 32.01,14.58 55.61,33.78 54.29,29.82 56.67,32.77 9.15,22.05 64.73,32.08 18.75,4.34 17.91,3.89 17.94,2.9 12.71,14.1 17.99,1.35 17.99,0.51 38.72,5.23 37.29,5.23 40.24,5.23 49.49,0.51 49.49,4.24 49.49,3.53 49.49,2.92 49.49,2.31 49.49,1.7 49.49,1.09 33.94,1.52 19.72,1.73 36.48,2.95 33.33,1.52 64.6,13.69 60.38,16.21 47.73,9.3 47.73,8.79 42.65,11.28 43.16,11.28 42.65,10.13 43.16,10.13 38.77,8.33 8.95,21.54 16.03,24.33 16.54,24.33 38.26,7.98 19.64,10.13 19.64,11.28 51.44,21.46 55.56,21.29 56.14,22.33 58.35,21.16 44.13,22.92 55.91,26.87 37.17,11.28 47.5,20.85 22.74,6.91 24.54,5.08 16.06,15.57 10.67,17.7 36.02,5.64 36.48,3.96 41.51,4.47 41.18,4.01 41.51,5.99 41.18,6.45 18.14,19.18 18.14,18.62 18.14,18.08 18.14,17.53 18.14,16.71 18.17,16.15 27.21,5.08 67.6,34.82 67.6,35.41 67.55,35.99 14.71,37.44 16.24,35.81 14.71,33.58 16.34,31.24 14.71,30.12 3.74,34.49 6.89,34.49 7.4,26.16 10.14,34.49 11.67,31.95 9.02,31.95 5.67,32.56 14.71,26.77 57.26,27.97 58.63,25.4 57.13,26.54 56.47,26.8 50.27,35.13 58.63,23.9 58.66,31.72 58.66,30.61 37.22,23.44 62.01,38.3 46.92,20.85 42.32,22.15 5.44,25.12 50.93,33.05 35.59,7.65 36.13,7.65 35.59,7.14 7.8,25.02 7.19,25.02 39.96,30.71 40.82,32.64 50.07,36.15 48.57,35.08 53.58,29.77 42.32,22.86 42.22,0.71 35.62,5.17 19.56,26.16 11.46,22.5 10.45,24.64 67.47,12.75 67.47,11.94 62.39,8.79 62.97,8.79 21.09,26.16 21.6,26.16 66.02,32.08 66.86,32.08 67.62,32.08 57.94,30.61 56.78,28.85
  pour Route2 (rank 4): 34.58,9.4 49.82,9.4 49.82,-0.46 34.58,-0.46
  pour Top (no thermals): 40.16,4.72 40.16,4.22 40.67,4.22 41.08,3.81 41.28,3.81 41.79,4.32 41.79,6.15 41.28,6.65 41.08,6.65 40.67,6.25 40.16,6.25 40.16,5.74 41.18,5.74 41.28,5.64 41.28,4.83 41.18,4.72
  cutout Bottom: 6.13,9.25 14.5,14.15 arc-70 17.51,12.41 20.28,7.63 arc-90 19.64,5.2 17.64,4.02 17.71,-0.28 12.36,-0.28 8.29,6.96 6.13,6.96
  cutout Top: 6.13,9.25 14.5,14.15 arc-70 17.51,12.41 20.28,7.63 arc-90 19.64,5.2 17.64,4.02 17.71,0.03 12.19,0.03 8.29,6.96 6.13,6.96
  cutout Route2: 6.13,9.25 14.5,14.15 arc-70 17.51,12.41 20.28,7.63 arc-90 19.64,5.2 17.64,4.02 17.71,-0.08 12.24,-0.08 8.29,6.96 6.13,6.96
  cutout Top: 34.17,-1.88 34.17,9.3 34.58,9.7 49.51,9.7 49.51,9.91 34.47,9.91 33.97,9.4 33.97,-2.08
  cutout Bottom: 34.17,-2.49 34.17,9.3 34.58,9.7 49.51,9.7 49.51,9.91 34.47,9.91 33.97,9.4 33.97,-2.69
  cutout Route15: 6.13,9.25 14.5,14.15 arc-70 17.51,12.41 20.28,7.63 arc-90 19.64,5.2 17.64,4.02 17.71,-0.18 12.3,-0.18 8.29,6.96 6.13,6.96
  pour Bottom (rank 4): 34.58,9.4 49.82,9.4 49.82,-0.66 34.58,-0.66
  pour Top (rank 4): 34.58,9.4 49.82,9.4 49.82,-0.36 34.58,-0.36
  cutout Bottom: 34.88,1.57 34.88,1.37 36.1,1.37 36.1,1.57
  cutout Bottom: 34.88,2.59 34.88,2.39 36.1,2.39 36.1,2.59
  cutout Bottom: 9.89,23.01 10.09,23.01 10.09,24.23 9.89,24.23
  cutout Bottom: 8.87,23.01 9.07,23.01 9.07,24.23 8.87,24.23
  pour Top (rank 6): -1.49,42.01 69.63,42.01 69.63,-1.17 -1.49,-1.17
  cutout Route2: 34.17,-2.08 34.17,9.3 34.58,9.7 49.51,9.7 49.51,9.91 34.47,9.91 33.97,9.4 33.97,-2.29
  pour Route2 (rank 6): -1.49,42.01 69.83,42.01 69.83,-1.37 -1.49,-1.37
  pour Bottom (rank 6): -1.49,42.01 70.24,42.01 70.24,-1.78 -1.49,-1.78
  cutout Top: 17.61,24.13 17.61,15.6 20.15,13.06 20.15,12.75 arc-90 20.05,12.65 arc-90 19.95,12.75 19.95,13.06 17.41,15.6 17.41,24.13 19.34,26.06 arc-90 19.44,26.06 arc-90 19.44,25.96
  cutout Bottom: 17.61,24.13 17.61,15.6 20.15,13.06 20.15,12.75 arc-90 20.05,12.65 arc-90 19.95,12.75 19.95,13.06 17.41,15.6 17.41,24.13 19.34,26.06 arc-90 19.44,26.06 arc-90 19.44,25.96
  cutout Route2: 17.61,24.13 17.61,23.16 17.41,23.16 17.41,24.13 19.34,26.06 arc-90 19.44,26.06 arc-90 19.44,25.96
GPIO0
  Top 0.203: U10.42 44.3,16.74 44.44,16.88 46.63,16.88 GPIO0.P$1
GPIO1
  Top 0.203: U10.43 45.8,17.24 46.46,17.91 GPIO1.P$1
GPIO2
  Top 0.203: U10.29 39.54,12.48 TP5.P$1
GPIO3
  Top 0.203: U10.28 39.04,12.52 TP6.P$1
LED_BLUE
  Top 0.203: U10.40 44.69,15.74 R13.2
LED_GREEN
  Top 0.203: U10.41 44.95,16.24 R12.2
LED_NRF_BLUE  (via drill 0.2)
  Top 0.203: U7.P23 v50.41,26.32 | R9.2 54.19,26.06 v54.06,26.06
  Bottom 0.203: v50.41,26.32 51.32,26.32 51.68,25.96 53.96,25.96 v54.06,26.06
LED_NRF_GREEN  (via drill 0.2)
  Top 0.203: v55.2,25.96 55.46,25.96 R8.2
  Bottom 0.203: U7.T23 50.57,25.8 50.74,25.96 51.25,25.96 51.55,25.65 54.9,25.65 v55.2,25.96
  other vias: 50.41,25.8
LED_NRF_RED  (via drill 0.2)
  Top 0.203: v56.36,25.76 56.83,25.76 R7.2 | U7.U24
  Bottom 0.203: v56.36,25.76 55.65,25.76 55.24,25.35 51.43,25.35 51.22,25.55 U7.U24
  other vias: 50.91,25.55
LED_RED
  Top 0.203: R11.2 44.89,14.43 44.07,15.24 U10.39
N$1
  Top 0.203: J1.B5 29.47,8.7 29.47,5.37 26.7,2.59 20.89,2.59 R19.1
N$2  (via drill 0.2)
  Top 0.305: Q2.B1 65.98,35.61 65.47,35.1 v65.46,35.1
  Top 0.406: D4.ANODE 65.77,33.96 65.54,34.19 v65.51,34.19 | v65.46,35.1 v64.93,35.1
  Bottom 0.406: LS1.- 64.43,30.71 65.51,31.79 v65.51,34.19 65.51,35.05 v65.46,35.1 v64.93,35.1
N$3
  Top 0.33: T1.1 26.3,12 U9.1
  pour Top: 32.39,12.04 32.39,11.94 arc90 32.42,11.91 32.42,12.04
N$4
  Top 0.33: C6.P$2 25.94,13.65 arc50 26.27,13.32 T1.3
N$5  (via drill 0.2)
  other vias: 13.65,17.32
N$6  (via drill 0.2)
  other vias: 13.65,16.51
N$7
  Top 0.33: C7.P$2 25.33,13.65 arc-50 25.01,13.32 T1.4
N$8
  Top 0.203: C25.1 21.51,14.54 21.53,14.53 R6.2
N$9
  cutout Top: 28.99,37.06 28.99,27.79 30.38,26.39 37.75,26.39 39.15,27.79 39.22,37.06
N$10
  cutout Bottom: 28.99,37.06 28.99,27.79 30.38,26.39 37.75,26.39 39.15,27.79 39.22,37.06
N$11
  Top 0.406: U5.4 23.83,29.13 C26.1
N$12
  Top 0.203: R27.2 18.8,18.75 18.8,17.91 C17.1
N$13
  Top 0.203: R18.1 20.63,3.81 21.55,2.9 25.53,2.9 26.62,3.98 J1.A5
N$14
  Top 0.203: U1.12 23.5,18.02 22.46,16.98 C16.1 22.46,15.42 R6.1
N$15
  Top 0.152: U7.H23 50.69,27.8 50.77,27.87 52.09,27.87 C2.1
  Top 0.33: C2.1 L1.2
N$16
  Top 0.203: U1.8 22.71,19.82 21.96,19.08 20,19.08 R27.1 19.82,18.8 C3.1
N$17
  cutout Route15: 56.17,28.09 58.91,27.23 58.91,26.18 56.17,27.04
  cutout Route2: 56.17,28.09 58.91,27.23 58.91,26.18 56.17,27.04
N$18
  Top 0.203: U7.B24 50.91,32.48 50.15,33.23 X3.3 49.18,33.93 C8.2
N$19
  Top 0.203: U7.A23 50.41,30.32 50.15,30.58 48.63,30.58 X3.1 47.26,31.95 C9.2
N$20
  cutout Bottom: 52.19,14.97 47.83,7.37 arc90 48.39,5.28 49.97,4.37 50.03,-0.66 55.61,-0.66 59.98,7.16 61.5,7.16 61.5,9.59
N$21
  Top 0.203: U1.5 20.4,21.02 20.15,21.27 19.19,21.27 18.75,20.84 R25.2
N$22
  Top 0.203: U10.44 44.8,17.74 R26.1
N$23  (via drill 0.2)
  Top 0.203: R12.1 50.43,16.31 51.34,17.22 52.25,17.22 TP7.P$1 53.47,15.9 57.44,13.56 v57.94,13.56 | D3.4 60.79,6.2 v60.79,6.25
  Route2 0.203: v57.94,13.56 59.34,13.56 59.85,13.06 61.65,13.06 62.87,11.84 64.09,11.84 64.34,11.58 64.34,8.69 61.91,6.25 v60.79,6.25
